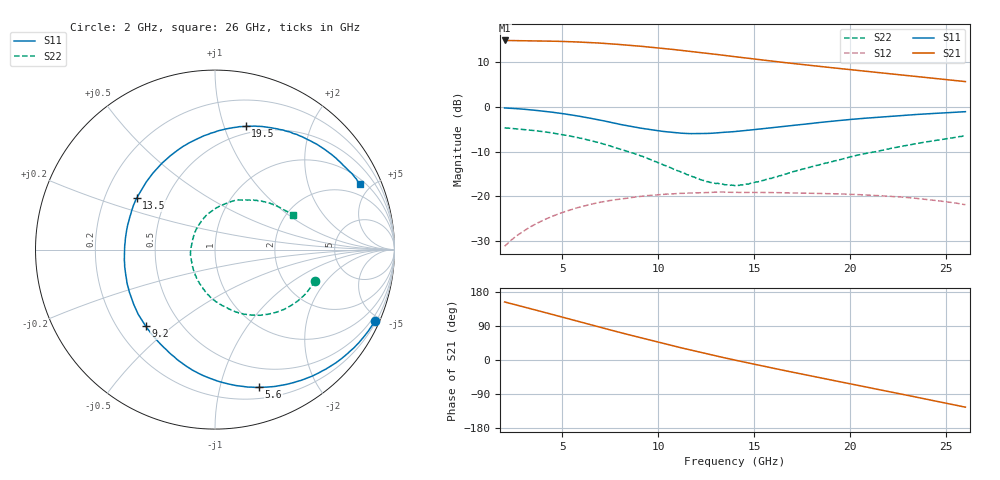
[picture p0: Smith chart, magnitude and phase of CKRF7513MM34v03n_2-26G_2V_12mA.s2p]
! CHUO DENSHI KOGYO Co.,Ltd.
! 22. July 2016
! CKRF7513MM34
! N-channel HJ-FET
! Vds = 2 V Id = 12 mA
# Hz S  MA  R 50
!	f	S11	S21	S12	S22
!	Hz	MAG	ANG	MAG	ANG	MAG	ANG	MAG	ANG
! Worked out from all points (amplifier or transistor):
!   241 points, 2 GHz to 26 GHz, reference 50 ohm
!   highest |S21| = 14.9 dB at 2 GHz (marker M1)
!   |S21| within 3 dB of that: start of sweep to 12.79 GHz
!   unconditionally stable (mu >= 1): 13.54 GHz to 20.12 GHz
!   at 6 GHz: K = 0.56, MSG = 18.4 dB, |S12| = -22.3 dB
!   at 14 GHz: K = 1.02, MAG = 14.3 dB, |S12| = -19.1 dB
!   at 26 GHz: K = 0.78, MSG = 13.8 dB, |S12| = -21.8 dB
!   lowest NFmin = 0.31 dB at 10 GHz
!   S11 on the Smith chart (normalised r, x): 2 GHz: 0.29, -4.66; 5.6 GHz: 0.30, -1.33; 9.2 GHz: 0.32, -0.40; 13.5 GHz: 0.34, +0.27; 19.5 GHz: 0.43, +1.18; 26 GHz: 1.28, +4.30
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2e9  0.9748 -24.1  5.535 153.2  0.02781 73.2  0.5837 -17.3
3e9  0.9422 -36.7  5.504 140.0  0.04125 65.6  0.561 -26.1
3.9e9  0.9024 -48.5  5.465 128.0  0.05276 58.6  0.5336 -34.4
4.8e9  0.8553 -60.7  5.413 115.9  0.06368 51.1  0.4996 -43.0
5.6e9  0.8061 -72.2  5.344 105.1  0.07256 44.4  0.4643 -51.0
6e9  0.7794 -78.1  5.303 99.7  0.07676 41.3  0.446 -55.1
6.7e9  0.7318 -89.1  5.211 90.2  0.08357 35.7  0.4099 -62.4
7.4e9  0.6828 -100.6  5.104 80.7  0.08937 30.0  0.3714 -70.3
8.1e9  0.6331 -112.6  4.962 71.4  0.09376 24.7  0.3319 -78.0
9.2e9  0.5748 -132.3  4.744 57.2  0.1007 17.0  0.2798 -91.9
1e10  0.5417 -147.9  4.572 47.0  0.1046 11.3  0.2378 -103.8
1.08e10  0.5176 -163.6  4.385 37.0  0.107 6.0  0.2019 -116.2
1.17e10  0.5034 178.9  4.172 26.1  0.1091 0.4  0.1695 -134.0
1.26e10  0.5057 162.2  3.96 15.6  0.1106 -4.8  0.1463 -154.2
1.35e10  0.5224 146.5  3.756 5.2  0.1116 -10.6  0.1348 -178.3
1.4e10  0.5312 138.6  3.641 -0.3  0.111 -13.2  0.1322 168.8
1.59e10  0.5853 112.9  3.262 -20.8  0.1104 -22.6  0.1591 126.8
1.8e10  0.6547 90.1  2.9 -42.4  0.1084 -32.6  0.2152 94.9
1.95e10  0.7078 76.1  2.682 -57.7  0.1065 -39.8  0.2585 78.0
2.2e10  0.7833 55.3  2.358 -83.1  0.1003 -52.1  0.3385 54.4
2.36e10  0.8277 42.4  2.18 -99.7  0.09462 -60.6  0.394 41.3
2.6e10  0.8856 24.2  1.922 -124.5  0.08101 -73.6  0.4761 24.2
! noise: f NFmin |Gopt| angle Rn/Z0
1e+10  0.31  0.466  97.3  0.07
1.05e+10  0.32  0.456  105.2  0.06
1.1e+10  0.35  0.425  112.7  0.06
1.15e+10  0.37  0.395  123.6  0.05
1.2e+10  0.39  0.375  134  0.04
1.25e+10  0.4  0.349  145.4  0.04
1.3e+10  0.43  0.333  157.5  0.04
1.35e+10  0.47  0.329  170.7  0.03
1.4e+10  0.49  0.331  -176.7  0.03
1.5e+10  0.52  0.356  -155  0.04
